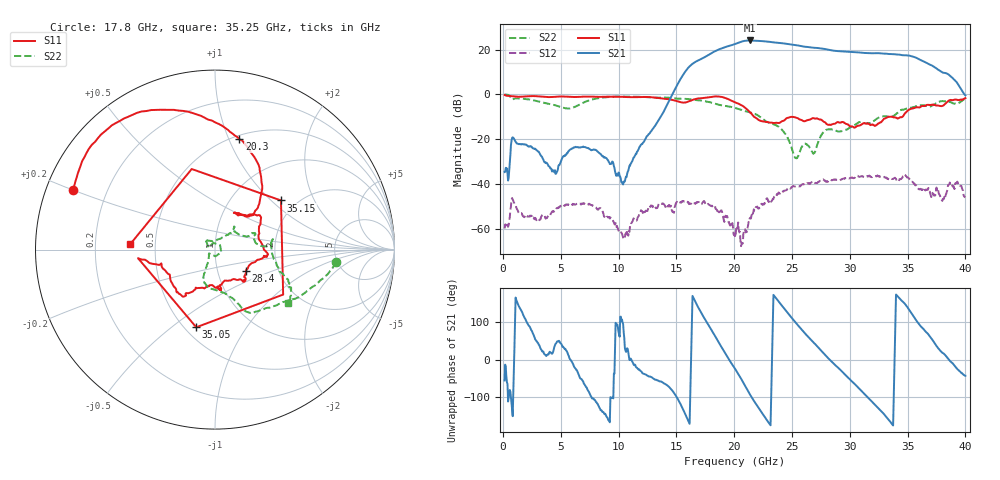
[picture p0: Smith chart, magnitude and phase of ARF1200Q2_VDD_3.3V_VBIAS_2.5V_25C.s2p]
!Bias:VDD=3.3V, VBIAS=2.5V
# GHz S DB R 50.0
!freq dBS11 angS11 dBS21 angS21 dBS12 angS12 dBS22 angS22
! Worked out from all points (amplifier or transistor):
!   798 points, 150 MHz to 40 GHz, reference 50 ohm
!   highest |S21| = 24.1 dB at 21.35 GHz (marker M1)
!   |S21| within 3 dB of that: 19.22 GHz to 26.46 GHz (7.237 GHz wide, 31.7 % of centre)
!   unconditionally stable (mu >= 1): start of sweep to end of sweep
!   at 6.8 GHz: K = 274.47, MAG = -14.7 dB, |S12| = -48.9 dB
!   at 20.1 GHz: K = 25.10, MAG = 26.3 dB, |S12| = -64.0 dB
!   at 40 GHz: K = 11.27, MAG = 9.3 dB, |S12| = -46.0 dB
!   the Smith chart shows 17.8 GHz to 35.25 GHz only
!   S11 on the Smith chart (normalised r, x): 17.8 GHz: 0.08, +0.20; 20.3 GHz: 0.54, +1.09; 28.4 GHz: 1.37, -0.34; 35.05 GHz: 0.57, -0.62; 35.15 GHz: 1.66, +1.15; 35.25 GHz: 0.36, +0.03
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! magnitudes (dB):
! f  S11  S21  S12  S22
! 150 MHz  -0.3  -34.7  -59.9  0.0
! 900 MHz  -0.9  -19.4  -47.4  -2.1
! 3.05 GHz  -0.9  -25.5  -56.4  -3.1
! 4.55 GHz  -1.0  -35.5  -51.3  -4.9
! 6.8 GHz  -1.0  -23.6  -48.9  -4.1
! 10.4 GHz  -1.1  -40.3  -64.0  -1.0
! 13.45 GHz  -1.6  -11.7  -49.3  -1.4
! 15.9 GHz  -3.5  11.1  -47.9  -2.0
! 17.8 GHz  -1.3  17.7  -49.3  -3.4
! 20.1 GHz  -3.6  22.6  -64.0  -6.1
! 20.3 GHz  -4.0  22.9  -59.6  -6.4
! 20.7 GHz  -5.0  23.7  -66.7  -7.1
! 21.35 GHz  -7.9  24.1  -55.3  -8.0
! 24 GHz  -12.5  22.9  -44.0  -15.1
! 25.3 GHz  -10.3  22.1  -41.1  -28.5
! 26.75 GHz  -10.7  20.9  -39.0  -25.6
! 28.4 GHz  -13.6  19.7  -38.3  -15.6
! 33.4 GHz  -10.0  18.1  -38.0  -10.1
! 35.05 GHz  -7.0  17.4  -37.2  -6.1
! 35.15 GHz  -6.8  17.3  -37.7  -6.0
! 35.25 GHz  -6.5  17.2  -38.3  -6.0
! 40 GHz  -1.6  -0.4  -46.0  -1.9
